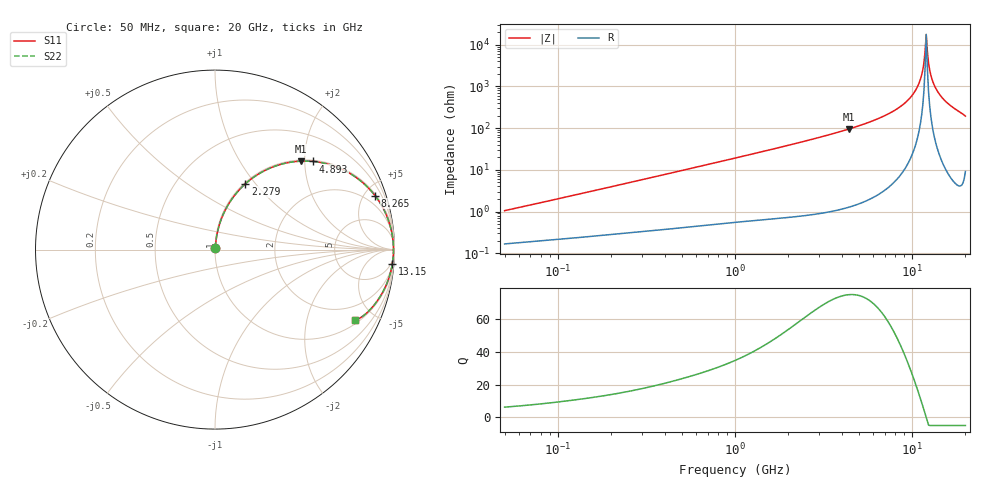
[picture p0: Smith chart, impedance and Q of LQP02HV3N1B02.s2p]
!Murata Part Number: LQP02HV3N1B02
!These Parameters are Measured in Series Mode Connection
!  o--[Z]--o
!Port1  Port2
!  o-------o
!Freq. Start=50[MHz] Stop=20[GHz], 401[Steps]
# Hz S RI R 50
!Freq.(Hz) S11(Real) S11(Imag) S21(Real) S21(Imag) S12(Real) S12(Imag) S22(Real) S22(Imag)
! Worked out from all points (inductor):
!   401 points, 50 MHz to 20 GHz, reference 50 ohm
!   read as one part in series: L = 3.25 nH near 51.52 MHz
!   highest Q = 75 at 4.406 GHz (marker M1), where L = 3.45 nH
!   self-resonance near 11.84 GHz
!   S11 on the Smith chart (normalised r, x): 50 MHz: 1.00, +0.02; 2.279 GHz: 1.02, +0.89; 4.893 GHz: 1.03, +2.20; 8.265 GHz: 1.12, +5.88; 13.15 GHz: 3, -25; 20 GHz: 1.18, -3.88
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5e7  0.00177 0.0103  0.9982 -0.0103  0.9982 -0.0103  0.00177 0.0103
1.364002e8  0.00313 0.0269  0.9969 -0.0269  0.9969 -0.0269  0.00313 0.0269
3.721004e8  0.00866 0.0709  0.9913 -0.0709  0.9913 -0.0709  0.00866 0.0709
1e9  0.0401 0.1823  0.9599 -0.1823  0.9599 -0.1823  0.0401 0.1823
2.279204e9  0.1695 0.3667  0.8305 -0.3667  0.8305 -0.3667  0.1695 0.3667
2.728004e9  0.2298 0.413  0.7702 -0.413  0.7702 -0.413  0.2298 0.413
4.405649e9  0.4776 0.4929  0.5224 -0.4929  0.5224 -0.4929  0.4776 0.4929
4.89267e9  0.5472 0.4911  0.4528 -0.4911  0.4528 -0.4911  0.5472 0.4911
7.442007e9  0.8323 0.3649  0.1677 -0.3649  0.1677 -0.3649  0.8323 0.3649
8.264682e9  0.8912 0.3011  0.1088 -0.3011  0.1088 -0.3011  0.8912 0.3011
9.600142e9  0.9555 0.1911  0.0445 -0.1911  0.0445 -0.1911  0.9555 0.1911
1.066139e10  0.983 0.1043  0.017 -0.1043  0.017 -0.1043  0.983 0.1043
1.115139e10  0.9898 0.0656  0.0102 -0.0656  0.0102 -0.0656  0.9898 0.0656
1.149051e10  0.9927 0.0394  0.00731 -0.0394  0.00731 -0.0394  0.9927 0.0394
1.166392e10  0.9936 0.0263  0.0064 -0.0263  0.0064 -0.0263  0.9936 0.0263
1.201863e10  0.9944 -3.92e-05  0.00564 3.92e-05  0.00564 3.92e-05  0.9944 -3.92e-05
1.238412e10  0.9937 -0.0264  0.00627 0.0264  0.00627 0.0264  0.9937 -0.0264
1.276073e10  0.9917 -0.0527  0.00831 0.0527  0.00831 0.0527  0.9917 -0.0527
1.314879e10  0.9883 -0.0789  0.0117 0.0789  0.0117 0.0789  0.9883 -0.0789
1.396067e10  0.9772 -0.1304  0.0228 0.1304  0.0228 0.1304  0.9772 -0.1304
1.527346e10  0.9506 -0.2047  0.0494 0.2047  0.0494 0.2047  0.9506 -0.2047
2e10  0.7796 -0.3916  0.2204 0.3916  0.2204 0.3916  0.7796 -0.3916
